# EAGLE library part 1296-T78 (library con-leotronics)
1.27mm SINGLE ROW FEMALE SOCKET Source: http://www.leotronics.co.uk/Conexcon/Data%20Sheets/sec.%20A/1296ing.pdf
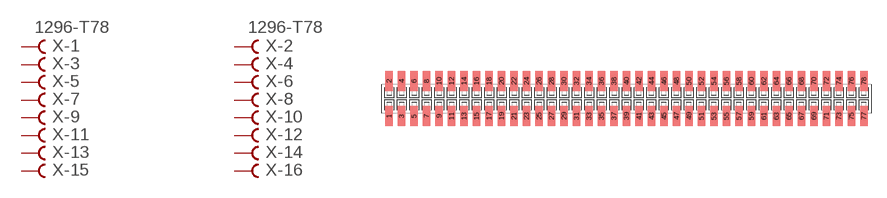
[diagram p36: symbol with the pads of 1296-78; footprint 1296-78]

Designator prefix X; gates -1=FVAL -2=FVAL -3=F -4=F -5=F -6=F -7=F -8=F -9=F -10=F -11=F -12=F -13=F -14=F -15=F -16=F -17=F -18=F -19=F -20=F -21=F -22=F -23=F -24=F -25=F -26=F -27=F -28=F -29=F -30=F -31=F -32=F -33=F -34=F -35=F -36=F -37=F -38=F -39=F -40=F -41=F -42=F -43=F -44=F -45=F -46=F -47=F -48=F -49=F -50=F -51=F -52=F -53=F -54=F -55=F -56=F -57=F -58=F -59=F -60=F -61=F -62=F -63=F -64=F -65=F -66=F -67=F -68=F -69=F -70=F -71=F -72=F -73=F -74=F -75=F -76=F -77=F -78=F

## 1296-T78 (OC_FARNELL: unknown; OC_NEWARK: unknown)  [1296-78]
1  -1:B  pas
2  -2:B  pas
3  -3:B  pas
4  -4:B  pas
5  -5:B  pas
6  -6:B  pas
7  -7:B  pas
8  -8:B  pas
9  -9:B  pas
10  -10:B  pas
11  -11:B  pas
12  -12:B  pas
13  -13:B  pas
14  -14:B  pas
15  -15:B  pas
16  -16:B  pas
17  -17:B  pas
18  -18:B  pas
19  -19:B  pas
20  -20:B  pas
21  -21:B  pas
22  -22:B  pas
23  -23:B  pas
24  -24:B  pas
25  -25:B  pas
26  -26:B  pas
27  -27:B  pas
28  -28:B  pas
29  -29:B  pas
30  -30:B  pas
31  -31:B  pas
32  -32:B  pas
33  -33:B  pas
34  -34:B  pas
35  -35:B  pas
36  -36:B  pas
37  -37:B  pas
38  -38:B  pas
39  -39:B  pas
40  -40:B  pas
41  -41:B  pas
42  -42:B  pas
43  -43:B  pas
44  -44:B  pas
45  -45:B  pas
46  -46:B  pas
47  -47:B  pas
48  -48:B  pas
49  -49:B  pas
50  -50:B  pas
51  -51:B  pas
52  -52:B  pas
53  -53:B  pas
54  -54:B  pas
55  -55:B  pas
56  -56:B  pas
57  -57:B  pas
58  -58:B  pas
59  -59:B  pas
60  -60:B  pas
61  -61:B  pas
62  -62:B  pas
63  -63:B  pas
64  -64:B  pas
65  -65:B  pas
66  -66:B  pas
67  -67:B  pas
68  -68:B  pas
69  -69:B  pas
70  -70:B  pas
71  -71:B  pas
72  -72:B  pas
73  -73:B  pas
74  -74:B  pas
75  -75:B  pas
76  -76:B  pas
77  -77:B  pas
78  -78:B  pas

## Footprint 1296-78 (pad centres in mm)
1.27mm SINGLE ROW FEMALE SOCKET Source: http://www.leotronics.co.uk/Conexcon/Data%20Sheets/sec.%20A/1296ing.pdf
smd 0.76 x 2.05: 1 -24.13,-1.78; 2 -24.13,1.78; 3 -22.86,-1.78; 4 -22.86,1.78; 5 -21.59,-1.78; 6 -21.59,1.78; 7 -20.32,-1.78; 8 -20.32,1.78; 9 -19.05,-1.78; 10 -19.05,1.78; 11 -17.78,-1.78; 12 -17.78,1.78; 13 -16.51,-1.78; 14 -16.51,1.78; 15 -15.24,-1.78; 16 -15.24,1.78; 17 -13.97,-1.78; 18 -13.97,1.78; 19 -12.7,-1.78; 20 -12.7,1.78; 21 -11.43,-1.78; 22 -11.43,1.78; 23 -10.16,-1.78; 24 -10.16,1.78; 25 -8.89,-1.78; 26 -8.89,1.78; 27 -7.62,-1.78; 28 -7.62,1.78; 29 -6.35,-1.78; 30 -6.35,1.78; 31 -5.08,-1.78; 32 -5.08,1.78; 33 -3.81,-1.78; 34 -3.81,1.78; 35 -2.54,-1.78; 36 -2.54,1.78; 37 -1.27,-1.78; 38 -1.27,1.78; 39 0,-1.78; 40 0,1.78; 41 1.27,-1.78; 42 1.27,1.78; 43 2.54,-1.78; 44 2.54,1.78; 45 3.81,-1.78; 46 3.81,1.78; 47 5.08,-1.78; 48 5.08,1.78; 49 6.35,-1.78; 50 6.35,1.78; 51 7.62,-1.78; 52 7.62,1.78; 53 8.89,-1.78; 54 8.89,1.78; 55 10.16,-1.78; 56 10.16,1.78; 57 11.43,-1.78; 58 11.43,1.78; 59 12.7,-1.78; 60 12.7,1.78; 61 13.97,-1.78; 62 13.97,1.78; 63 15.24,-1.78; 64 15.24,1.78; 65 16.51,-1.78; 66 16.51,1.78; 67 17.78,-1.78; 68 17.78,1.78; 69 19.05,-1.78; 70 19.05,1.78; 71 20.32,-1.78; 72 20.32,1.78; 73 21.59,-1.78; 74 21.59,1.78; 75 22.86,-1.78; 76 22.86,1.78; 77 24.13,-1.78; 78 24.13,1.78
